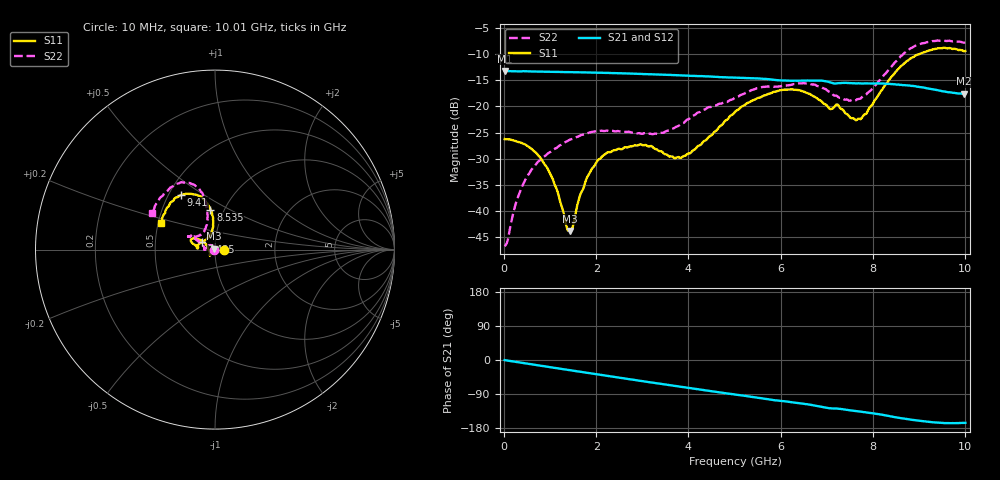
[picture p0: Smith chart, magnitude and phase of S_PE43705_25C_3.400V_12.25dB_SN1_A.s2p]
! Device ID: PE43705
! Serial: 1
! Insertion: A
! Impedance: 50 ohm
! Temp: 25C
! VDD: 3.400V
! Attenuation Step: 12.25dB
#  Hz  S  RI  R  50
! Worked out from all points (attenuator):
!   401 points, 10 MHz to 10.01 GHz, reference 50 ohm
!   highest |S21| = -13.24 dB at 10 MHz (marker M1); lowest = -17.6 dB at 9.985 GHz (marker M2)
!   lowest |S11| = -43.8 dB at 1.435 GHz (marker M3), VSWR 1.01, Z = 49.6 + j0.466 ohm
!   |S11| at or under -10 dB: start of sweep to 9.017 GHz
!   |S22| runs from -46.7 to -7.4 dB; largest |S21 - S12| = 0.0017
!   S11 on the Smith chart (normalised r, x): 10 MHz: 1.10, +0.00; 7.435 GHz: 0.86, +0.07; 8.535 GHz: 0.86, +0.40; 9.41 GHz: 0.58, +0.41; 10.01 GHz: 0.51, +0.17
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1e7  0.0488 0.000118  0.2177 -0.000956  0.2179 -0.000918  -0.00462 0.000411
2.85e8  0.0453 0.00777  0.2152 -0.0208  0.2152 -0.0207  -0.00561 0.0119
5.35e8  0.0386 0.0141  0.2122 -0.0388  0.2123 -0.0386  -0.0105 0.02
9.85e8  0.0178 0.0151  0.2028 -0.0689  0.2028 -0.0688  -0.0268 0.0247
1.36e9  -0.000614 0.00694  0.1918 -0.0921  0.1919 -0.092  -0.0413 0.0209
1.435e9  -0.00445 0.0047  0.1892 -0.0966  0.1892 -0.0964  -0.0441 0.0197
1.685e9  -0.015 -0.00384  0.1798 -0.1108  0.1799 -0.1107  -0.0515 0.0143
1.885e9  -0.0222 -0.0106  0.1716 -0.1217  0.1717 -0.1214  -0.056 0.00979
2.21e9  -0.0273 -0.0227  0.1568 -0.1379  0.1569 -0.1377  -0.0586 0.00257
2.935e9  -0.0293 -0.0317  0.1185 -0.1668  0.1188 -0.1667  -0.0555 0.00253
3.36e9  -0.0267 -0.0264  0.0938 -0.1781  0.094 -0.1778  -0.0546 0.00622
3.885e9  -0.0331 -0.00434  0.0624 -0.1872  0.0625 -0.1871  -0.0662 0.0205
5.01e9  -0.0733 0.05  -0.00362 -0.1878  -0.00332 -0.1881  -0.1068 0.0569
5.985e9  -0.1288 0.0609  -0.0538 -0.1689  -0.0531 -0.1692  -0.1363 0.0743
6.685e9  -0.1226 0.0325  -0.0854 -0.1543  -0.0853 -0.1542  -0.1449 0.0719
7.435e9  -0.0743 0.0404  -0.1111 -0.1252  -0.1105 -0.1256  -0.0818 0.0831
7.785e9  -0.033 0.0734  -0.1211 -0.1125  -0.1209 -0.1132  -0.057 0.1108
8.36e9  -0.0112 0.1806  -0.1393 -0.0869  -0.1385 -0.0873  -0.0445 0.2248
8.535e9  -0.0256 0.2216  -0.1423 -0.0761  -0.1417 -0.0775  -0.0553 0.2716
9.41e9  -0.1878 0.3049  -0.1382 -0.036  -0.1374 -0.0357  -0.2187 0.3655
9.985e9  -0.2965 0.1574  -0.128 -0.032  -0.1286 -0.0321  -0.3441 0.2143
1.001e10  -0.3035 0.1485  -0.1286 -0.0324  -0.129 -0.0323  -0.3519 0.2032
